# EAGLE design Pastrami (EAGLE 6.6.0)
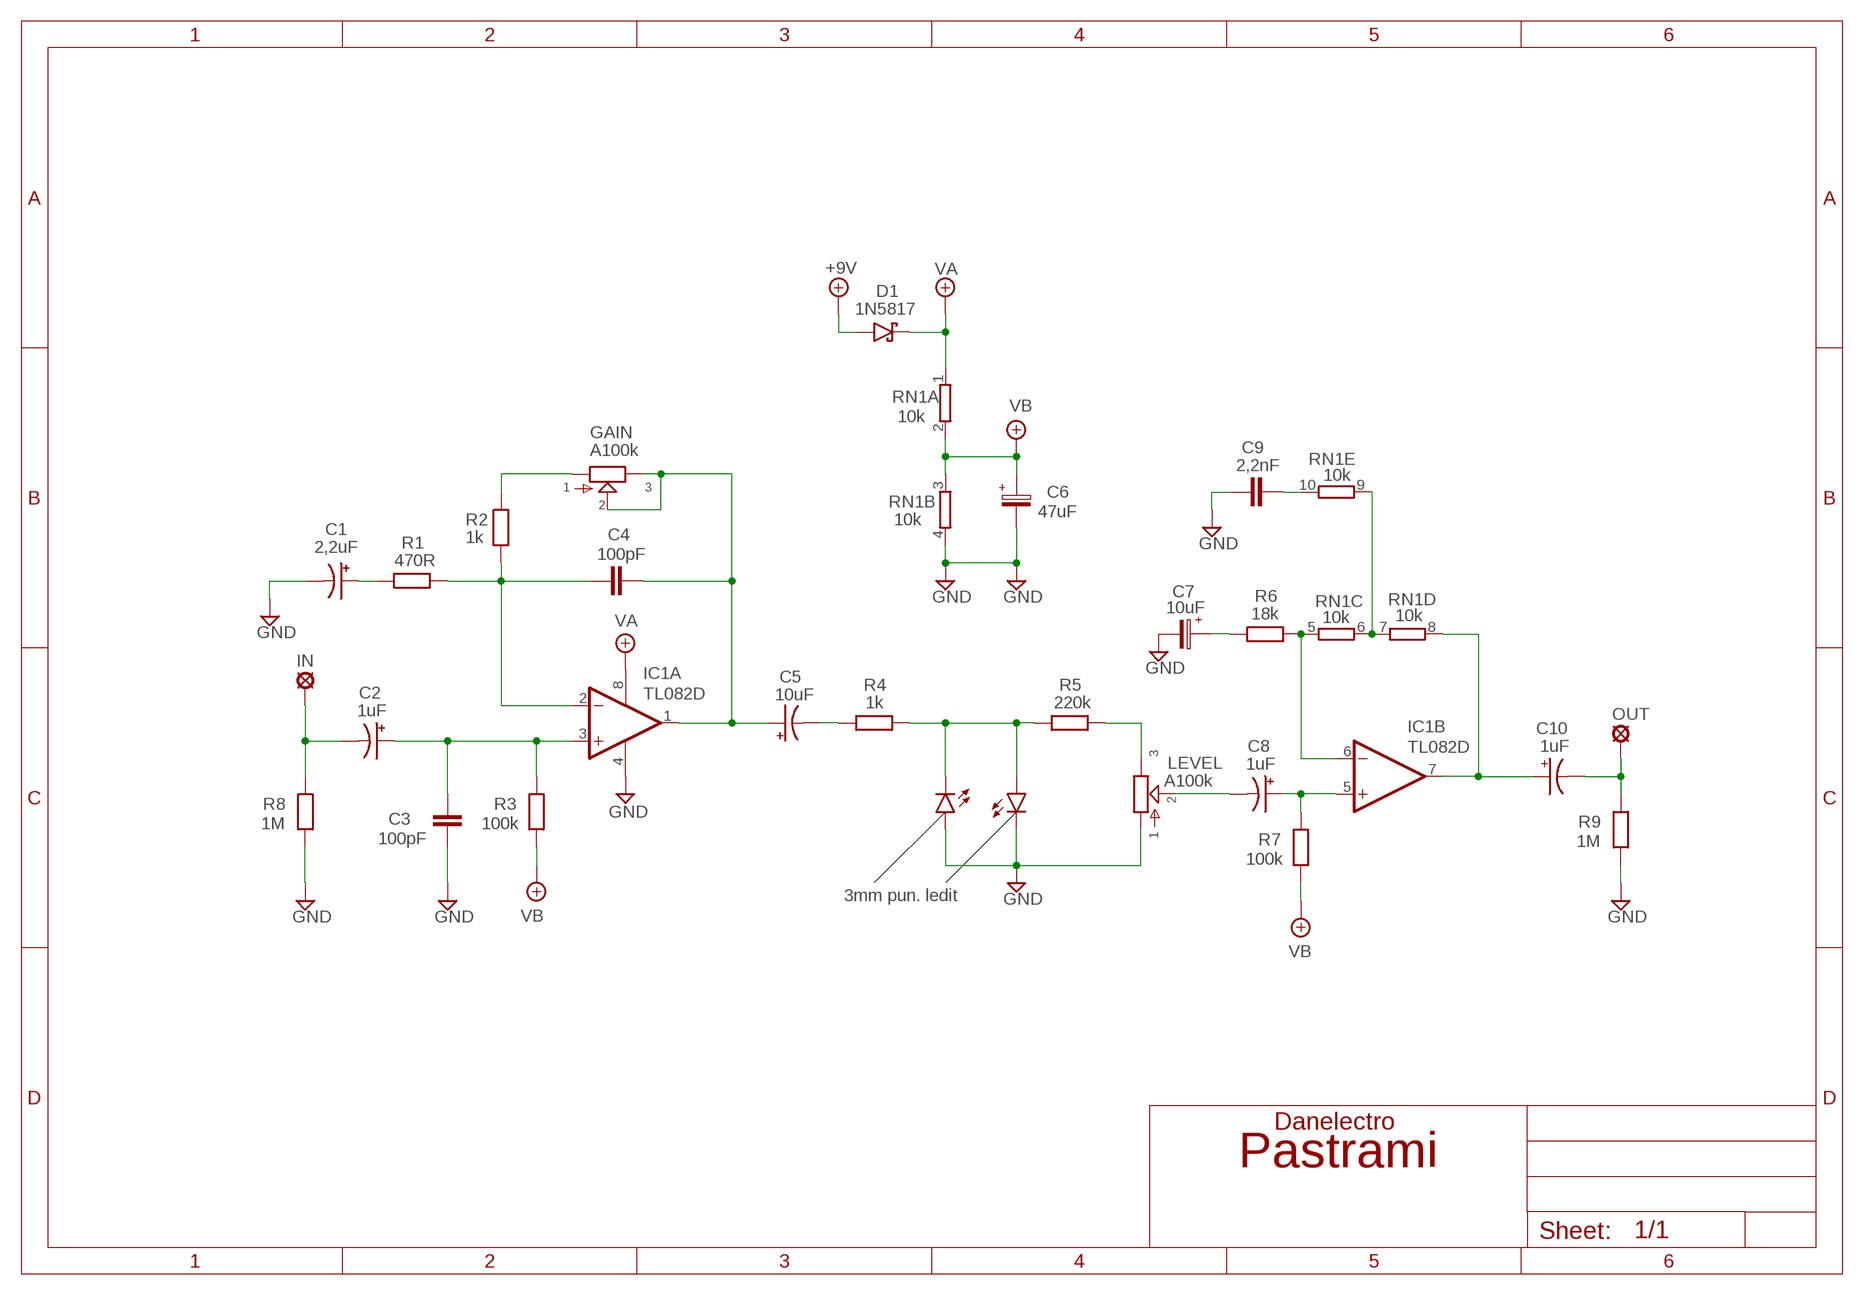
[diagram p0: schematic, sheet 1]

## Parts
+9V  +9V  +9V(T)1  [ROUND]
C1  2,2uF  044A1  [044A]
C2  1uF  044A1  [044A]
C3  100pF  050X030_0251  [050X030_025]
C4  100pF  050X030_0251  [050X030_025]
C5  10uF  044A2  [044A_2]
C6  47uF  063-EU  [063_025]
C7  10uF  063-EU  [063_025]
C8  1uF  044A1  [044A]
C9  2,2nF  1NF-15NF  [3,5MM]
C10  1uF  044A1  [044A]
D1  1N5817  [DO41-3]
D2  LED3MM  [LED3MM]
D3  3mm pun. ledit  LED3MM  [LED3MM]
GAIN  A100k  POT-EU16MM  [16MM]
GND  GND  GND(T)1  [ROUND]
GND5  GND  GND(T)1  [ROUND]
IC1  TL082D  [SO08]
IN  MCS10B  [MCS10B]
LEVEL  A100k  POT-EU16MM  [16MM]
OUT  MCS10B  [MCS10B]
R1  470R  6MM-EU3  [R0207/3]
R2  1k  6MM-EU3  [R0207/3]
R3  100k  6MM-EU3  [R0207/3]
R4  1k  6MM-EU3  [R0207/3]
R5  220k  6MM-EU3  [R0207/3]
R6  18k  6MM-EU3  [R0207/3]
R7  100k  6MM-EU3  [R0207/3]
R8  1M  6MM-EU3  [R0207/3]
R9  1M  6MM-EU3  [R0207/3]
RN1  10k  E5R  [SIL10]

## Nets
+9V: +9V.1(+9V) D1.A
GND: C1.2(-) C3.1 C6.- C7.- C9.1 D2.A D3.K(C) GND5.1(GND) GND.1(GND) IC1.4(P:V-) LEVEL.1 R8.1 R9.1 RN1.4
N$1: C2.1(+) C3.2 IC1.3(A:+IN) R3.2
N$2: C2.2(-) IN.MP R8.2
N$3: C4.1 C5.1(+) GAIN.2 GAIN.3 IC1.1(A:OUT)
N$4: GAIN.1 R2.2
N$5: C4.2 IC1.2(A:-IN) R1.1 R2.1
N$6: C5.2(-) R4.2
N$7: D2.K(C) D3.A R4.1 R5.2
N$8: LEVEL.3 R5.1
N$9: C8.2(-) LEVEL.2
N$10: C8.1(+) IC1.5(B:+IN) R7.2
N$11: RN1.6 RN1.7 RN1.9
N$12: C10.1(+) IC1.7(B:OUT) RN1.8
N$13: IC1.6(B:-IN) R6.1 RN1.5
N$14: C1.1(+) R1.2
N$15: C9.2 RN1.10
N$16: C7.+ R6.2
N$17: C10.2(-) OUT.MP R9.2
VA: D1.C IC1.8(P:V+) RN1.1
VB: C6.+ R3.1 R7.1 RN1.2 RN1.3

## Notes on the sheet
- Danelectro

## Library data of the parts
+9V = gm-supply:+9V(T): +9V Voltage Supply
C1 C2 C5 C8 C10 = Tantaalit:044A: .1 - 1.5µF
C3 C4 = Keraamiset kondensaattorit:050X030_025: 47 - 120pF
C6 C7 = Elektrolyytit:063-EU
C9 = Mylar Kondensaattorit:1NF-15NF: 1nF-15nF
D1 = Diodit:1N5817
D2 D3 = Diodit:LED
GAIN LEVEL = gm-pots:POT-EU
GND GND5 = gm-supply:GND(T): Ground
IC1 = Operaatiovahvistimet:TL082: OP AMP
IN OUT = Padit:MCS10B: SOLDER PAD
R1-R9 = Vastukset:6MM-EU: 6mm Resistors (European schematic symbol)
RN1 = resistor-sil:E5R: SIL RESISTOR; OC_FARNELL: unknown; OC_NEWARK: unknown

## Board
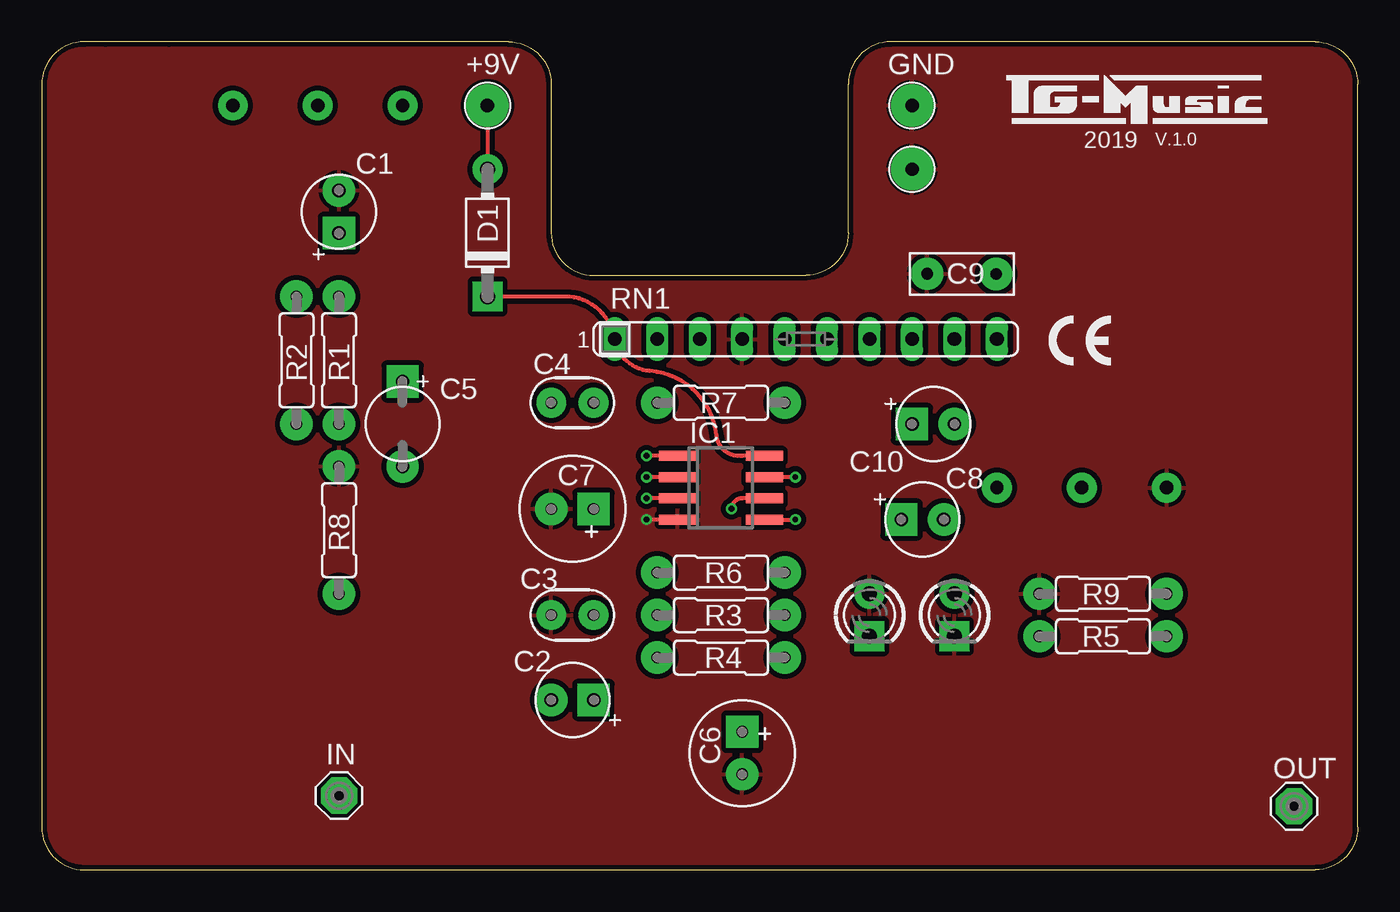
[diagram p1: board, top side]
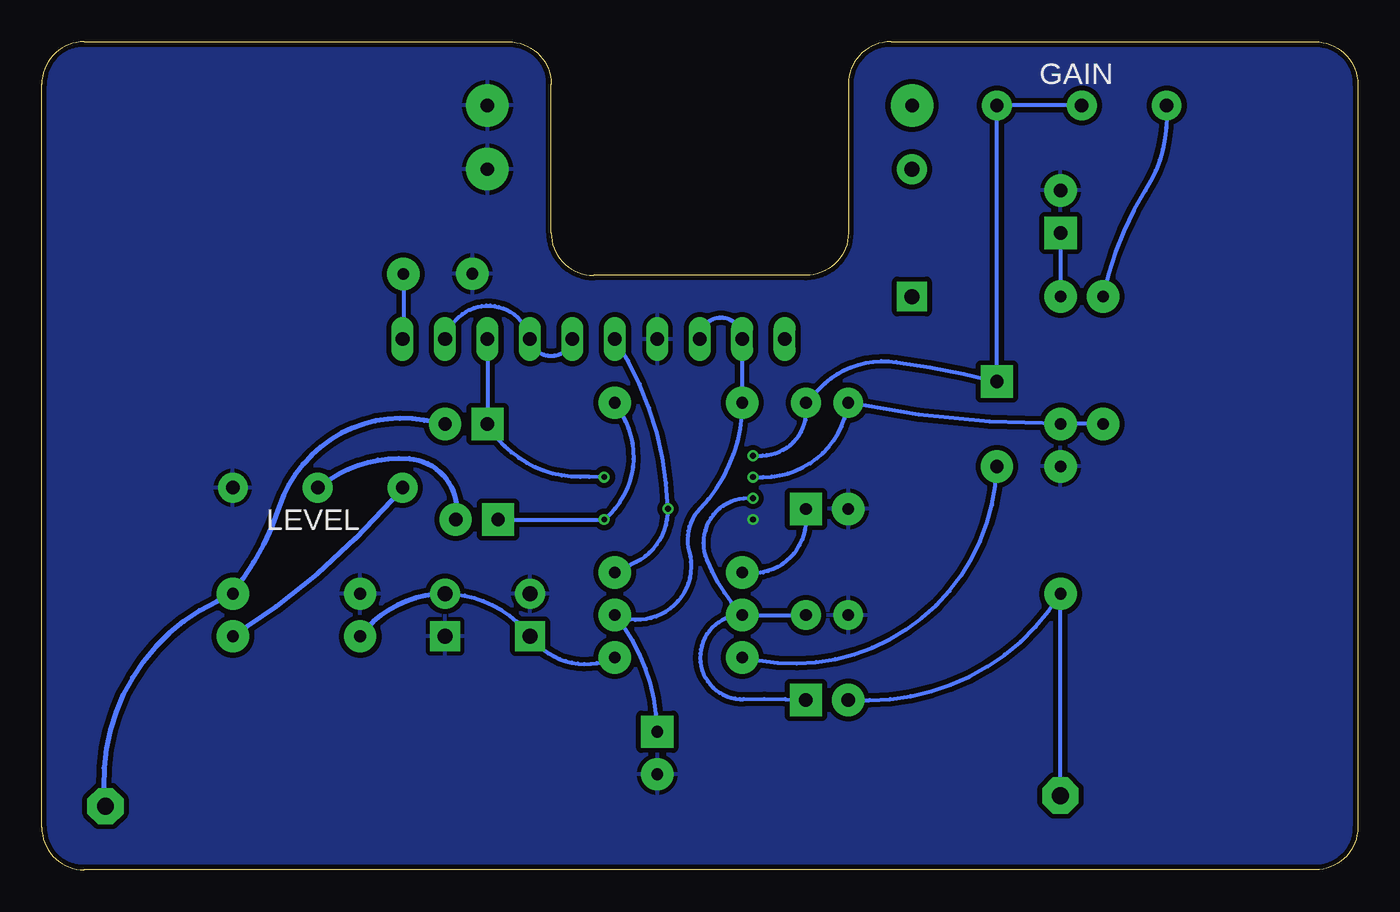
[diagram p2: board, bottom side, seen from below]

Size 78.74 x 49.53 mm. Coordinates in mm from the lower left corner, seen from the top.
Outline: 7.62,49.53 3.81,49.53
Outline: 78.74,2.54 78.74,46.99 arc90 76.2,49.53 50.8,49.53 arc90 48.26,46.99 48.26,38.1 arc-90 45.72,35.56 33.02,35.56 arc-90 30.48,38.1 30.48,46.99 arc90 27.94,49.53 2.54,49.53 arc90 0,46.99 0,2.54 arc90 2.54,0 76.2,0 arc90 78.74,2.54
Copper layers (1*16): Top 0.035mm / dielectric 1.5mm / Bottom 0.035mm
Design rules "ITEADstudio": minimum track width 10mil, minimum drill 12mil, track to track 12mil, track to pad 12mil, pad to pad 12mil, via to via 12mil, smd to smd 0mil, copper to edge 12mil, drill to drill 12mil, minimum pad ring 10mil, minimum via ring 6mil, stop-mask expansion 4mil, vias tented up to drill 100mil, thermal gap 10mil

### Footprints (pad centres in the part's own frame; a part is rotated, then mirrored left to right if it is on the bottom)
ROUND = drill 0.8 pad 2.54: 1 0,0
044A = drill 0.8 pad 1.93 square: 1 -1.27,0 | drill 0.8 pad 1.93: 2 1.27,0
050X030_025 = drill 0.7 pad 1.778: 1 -1.27,0; 2 1.27,0
044A_2 = drill 0.8 pad 1.93 square: 1 -2.54,0 | drill 0.8 pad 1.93: 2 2.54,0
063_025 = drill 0.7 pad 1.93 square: + -1.27,0 | drill 0.7 pad 1.93: - 1.27,0
3,5MM = drill 0.7 pad 1.93: 1 -1.905,0; 2 2.221,-0.016
DO41-3 = drill 0.9 pad 1.778: A 3.81,0 | drill 0.9 pad 1.778 square: C -3.81,0
LED3MM = drill 0.9 pad 1.778: A -1.27,0 | drill 0.9 pad 1.778 square: K 1.27,0
16MM = drill 0.8 pad 1.778: 1 5.08,0; 2 0,0; 3 -5.08,0
SO08 = smd 0.6 x 2.2: 1 -1.905,-2.6; 2 -0.635,-2.6; 3 0.635,-2.6; 4 1.905,-2.6; 5 1.905,2.6; 6 0.635,2.6; 7 -0.635,2.6; 8 -1.905,2.6
MCS10B = drill 1.016 pad 2.159 octagon: MP 0,0
R0207/3 = drill 0.7 pad 1.93: 1 -3.81,0; 2 3.81,0
SIL10 = drill 0.813 long: 1 -11.43,0; 2 -8.89,0; 3 -6.35,0; 4 -3.81,0; 5 -1.27,0; 6 1.27,0; 7 3.81,0; 8 6.35,0; 9 8.89,0; 10 11.43,0

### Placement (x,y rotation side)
+9V  26.67,45.72 0 top
C1  17.78,39.37 90 top
C2  31.75,10.16 180 top
C3  31.75,15.24 0 top
C4  31.75,27.94 180 top
C5  21.59,26.67 270 top
C6  41.91,6.99 270 top
C7  31.75,21.59 180 top
C8  52.7,20.95 0 top
C9  54.88,35.65 0 top
C10  53.34,26.67 0 top
D1  26.67,38.1 90 top
D2  49.53,15.24 270 top
D3  54.61,15.24 270 top
GAIN  16.51,45.72 0 bottom
GND  52.07,45.72 0 top
GND5  52.07,41.91 0 top
IC1  40.64,22.86 270 top
IN  17.78,4.45 0 top
LEVEL  62.23,22.86 180 bottom
OUT  74.93,3.81 0 top
R1  17.78,30.48 90 top
R2  15.24,30.48 90 top
R3  40.64,15.24 180 top
R4  40.64,12.7 180 top
R5  63.5,13.97 180 top
R6  40.64,17.78 180 top
R7  40.64,27.94 0 top
R8  17.78,20.32 270 top
R9  63.5,16.51 0 top
RN1  45.72,31.75 0 top

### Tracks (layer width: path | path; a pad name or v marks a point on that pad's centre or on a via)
+9V
  Top 0.254: +9V.1 D1.A
GND  (via drill 0.35)
  Top 0.254: IC1.4 v36.2,20.95
  pour Bottom: 0,2.54 0,46.99 arc-90 2.54,49.53 27.94,49.53 arc-90 30.48,46.99 30.48,38.1 arc90 33.02,35.56 45.72,35.56 arc90 48.26,38.1 48.26,46.99 arc-90 50.8,49.53 76.2,49.53 arc-90 78.74,46.99 78.74,2.54 arc-90 76.2,0 2.54,0 arc-90
  pour Top: 0,2.54 0,46.99 arc-90 2.54,49.53 27.94,49.53 arc-90 30.48,46.99 30.48,38.1 arc90 33.02,35.56 45.72,35.56 arc90 48.26,38.1 48.26,46.99 arc-90 50.8,49.53 76.2,49.53 arc-90 78.74,46.99 78.74,2.54 arc-90 76.2,0 2.54,0 arc-90
N$1  (via drill 0.35)
  Top 0.254: IC1.3 v36.2,22.23
  Bottom 0.254: R3.2 C3.2 | R3.2 arc-182 36.74,10.21 arc5 C2.1 | v36.2,22.23 36.48,22.23 arc-113 38.95,18.53 arc-19 37.01,15.41 R3.2
N$2
  Bottom 0.254: IN.MP R8.2 arc58 29.21,10.16 C2.2
N$3  (via drill 0.35)
  Top 0.254: IC1.1 v36.2,24.77
  Bottom 0.254: GAIN.2 GAIN.3 C5.1 arc-6 27.61,30.37 arc-54 32.21,28.79 C4.1 arc98 35.61,24.78 v36.2,24.77
N$4
  Bottom 0.254: GAIN.1 11.43,45.09 arc32 12.7,40.64 arc-20 R2.2
N$5  (via drill 0.35)
  Top 0.254: IC1.2 v36.2,23.5
  Bottom 0.254: R2.1 R1.1 arc11 C4.2 arc82 35.56,23.5 v36.2,23.5
N$6
  Bottom 0.254: R4.2 35.87,12.53 arc-98 C5.2
N$7
  Bottom 0.254: D3.A arc53 D2.K arc-78 R4.1
  Bottom 0.305: D3.A arc-53 R5.2
N$8
  Bottom 0.305: LEVEL.3 57.8,22.11 arc17 R5.1
N$9
  Bottom 0.305: LEVEL.2 61.49,23.35 arc38 56.75,24.59 arc96 C8.2
N$10  (via drill 0.35)
  Top 0.254: IC1.5 v45.09,20.95
  Bottom 0.254: C8.1 v45.09,20.95 arc-80 44.03,27.23 R7.2
N$11
  Bottom 0.254: RN1.9 54.37,32.26 arc142 RN1.7 arc-154 RN1.6
N$12  (via drill 0.35)
  Top 0.254: v45.09,23.5 IC1.7
  Bottom 0.254: v45.09,23.5 45.98,23.5 46.51,23.5 arc60 C10.1 RN1.8
N$13  (via drill 0.35)
  Top 0.254: IC1.6 41.91,22.23 arc90 v41.27,21.59
  Bottom 0.254: R6.1 43.18,18.41 arc-65 v41.27,21.59 arc-32 RN1.5
N$14
  Bottom 0.254: C1.1 R1.2
N$15
  Bottom 0.254: C9.2 57.1,31.8 arc90 RN1.10
N$16
  Bottom 0.254: C7.+ 33.02,20.95 arc100 R6.2
N$17
  Bottom 0.305: R9.2 67.48,16.43 | 67.48,16.43 68.28,16.05 arc-72 OUT.MP | C10.2 55.85,26.89 arc-82 64.53,21.72 arc22 67.48,16.43
VA
  Top 0.254: IC1.8 41.91,24.77 arc-91 40.37,25.99 arc80 36.39,29.84 arc-77 RN1.1 arc81 31.29,34.29 D1.C
VB
  Bottom 0.254: C6.+ 41.92,8.4 arc-39 R3.1 arc-130 40.01,19.05 arc59 39.37,21.59 arc-44 R7.1 RN1.2 arc-180 RN1.3

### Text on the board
tNames: 2019 | V.1.0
